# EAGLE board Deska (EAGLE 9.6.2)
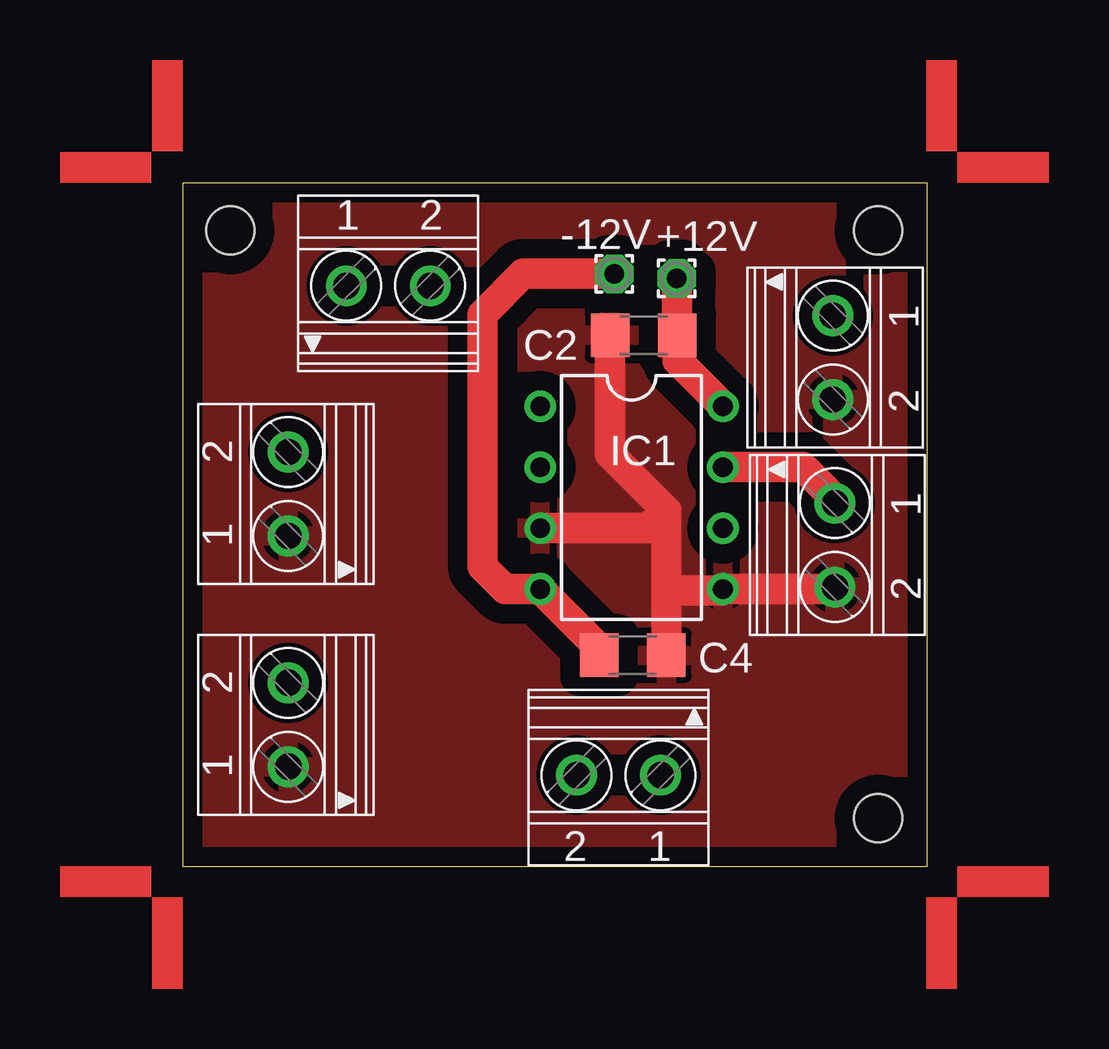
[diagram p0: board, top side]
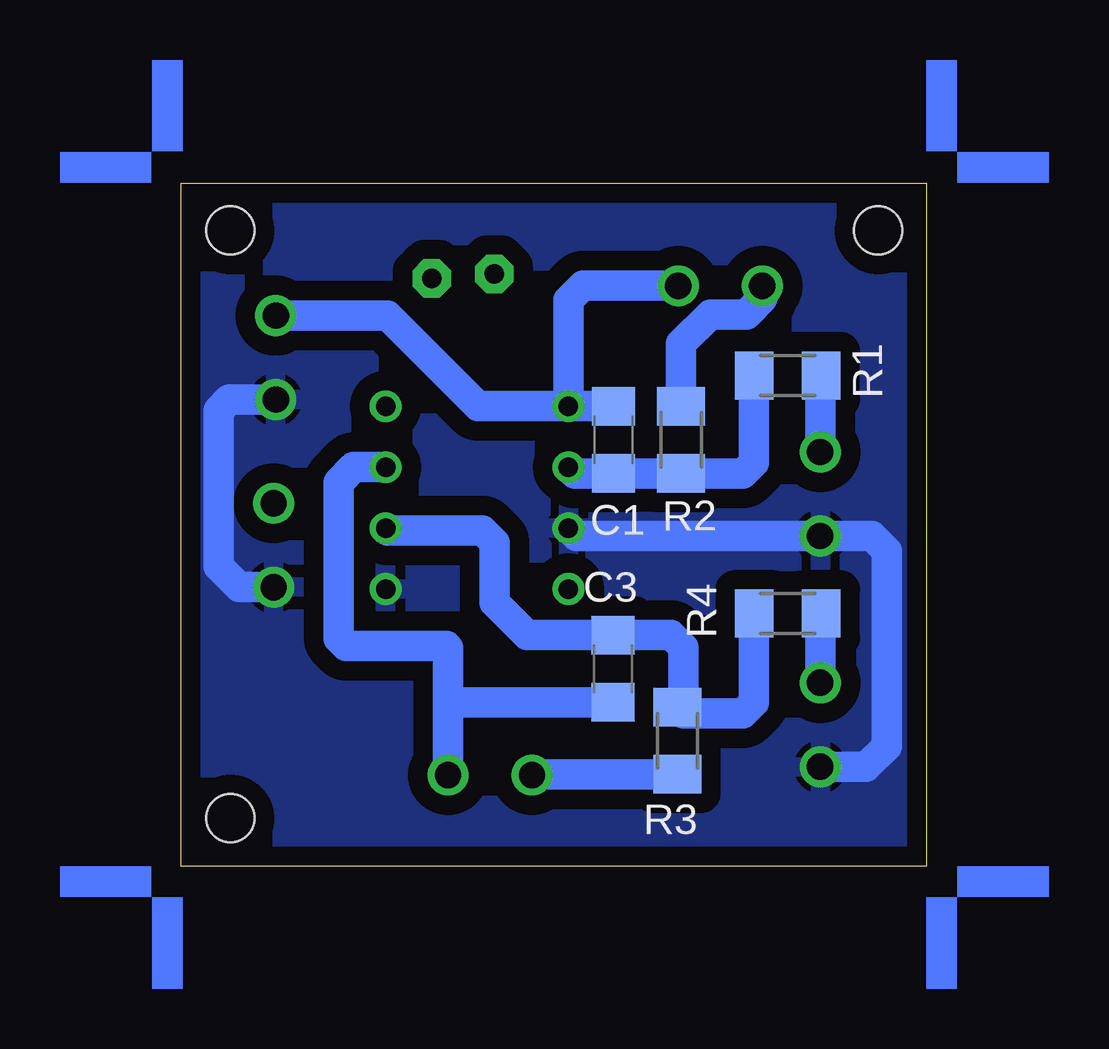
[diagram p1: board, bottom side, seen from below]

Size 31.05 x 28.48 mm. Coordinates in mm from the lower left corner, seen from the top.
Outline: 0,0 31.05,0 31.05,28.48 0,28.48 0,0
Copper layers (1*16): Top 0.035mm / dielectric 1.5mm / Bottom 0.035mm
Design rules "default *": minimum track width 6mil, minimum drill 0.35mm, track to track 6mil, track to pad 6mil, pad to pad 6mil, via to via 6mil, smd to smd 6mil, copper to edge 20mil, drill to drill 6mil, minimum pad ring 10mil, minimum via ring 8mil, stop-mask expansion 4mil, vias tented up to drill 0mil, thermal gap 10mil
Holes 2 mm at 2,26.5 29,2 29,26.5

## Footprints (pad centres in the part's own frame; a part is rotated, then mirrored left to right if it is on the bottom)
1,6/0,8 = drill 0.813 pad 1.6 octagon: 1 0,0
C1206 = smd 1.6 x 1.8: 1 -1.4,0; 2 1.4,0
DIL08 = drill 0.813 pad 1.27: 1 -3.81,-3.81; 2 -1.27,-3.81; 3 1.27,-3.81; 4 3.81,-3.81; 5 3.81,3.81; 6 1.27,3.81; 7 -1.27,3.81; 8 -3.81,3.81
M1206 = smd 1.6 x 2: 1 -1.4,0; 2 1.4,0
1751248 = drill 1.1 pad 1.7: 1 -1.75,-0.1; 2 1.75,-0.1

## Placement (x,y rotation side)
+12V  [1,6/0,8]  20.61,24.5 270 top
-12V  [1,6/0,8]  18,24.69 0 top
C1  [C1206]  13.03,17.77 90 bottom
C2  [C1206]  19.23,22.13 180 top
C3  [C1206]  13.05,8.23 270 bottom
C4  [C1206]  18.77,8.79 0 top
IC1  NE5532  [DIL08]  18.72,15.36 270 top
R1  [M1206]  5.77,20.45 180 bottom
R2  [M1206]  10.21,17.77 90 bottom
R3  [M1206]  10.37,5.23 270 bottom
R4  [M1206]  5.77,10.53 180 bottom
U$1  [ANGLE-SW1-16]  31,28.5 0 top
U$2  [ANGLE-SW1-16]  0,28.5 90 top
U$3  [ANGLE-SW1-16]  0,0 180 top
U$4  [ANGLE-SW1-16]  31,0 270 top
X1  1751248  [1751248]  27.21,21.2 270 top
X2  1751248  [1751248]  27.3,13.38 270 top
X3  1751248  [1751248]  4.31,15.51 90 top
X4  1751248  [1751248]  4.31,5.89 90 top
X5  1751248  [1751248]  8.58,24.29 0 top
X6  1751248  [1751248]  18.18,3.69 180 top

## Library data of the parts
+12V -12V = wirepad
C1-C4 = rcl; SPICEPREFIX: C
IC1 = linear
R1-R4 = rcl; SPICEPREFIX: R
U$1-U$4 = marks
X1-X6 = con-phoenix-350; OC_FARNELL: unknown; OC_NEWARK: unknown

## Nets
+12V: +12V.1 C2.1 IC1.8
-12V: -12V.1 C4.1 IC1.4
GND: C2.2 C4.2 IC1.3 IC1.5 X1.2 X2.2 X3.1 X4.1
N$1: C1.1 IC1.2 R1.2 R2.1
N$2: C3.1 IC1.6 R3.1 R4.2
N$3: R2.2 X5.1
N$4: R3.2 X6.2
N$5: C1.2 IC1.1 X1.1 X5.2
N$6: C3.2 IC1.7 X2.1 X6.1
N$7: R1.1 X3.2
N$8: R4.1 X4.2

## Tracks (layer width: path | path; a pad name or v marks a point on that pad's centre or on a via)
+12V
  Top 1.27: IC1.8 20.63,21.07 C2.1 20.61,22.15 +12V.1
-12V
  Top 1.27: C4.1 17.37,9.09 IC1.4 13.45,11.55 12.5,12.5 12.5,23 14.19,24.69 -12V.1
GND
  Top 1.27: C2.2 17.83,17.17 20.17,14.83 | 20.17,14.83 20.17,11.5 | 20.17,11.5 C4.2 | 20.17,11.5 22.48,11.5 IC1.5 27.12,11.55 X2.2 | IC1.3 19.43,14.09 20.17,14.83
  Bottom 1.27: X4.1 2.5,4.14 1.64,5 1.64,13.14 2.26,13.76 X3.1 14.58,13.76 IC1.3 | X1.2 29.05,19.45 29.5,19 29.5,12.5 28.63,11.63 X2.2
  pour Top (isolate 0.813): 0,0 31,0 31,28.5 0,28.5
  pour Bottom (isolate 0.813): 0,0 31,0 31,28.5 0,28.5
N$1
  Bottom 1.27: R1.2 7.17,16.83 7.63,16.37 R2.1 C1.1 14.65,16.37 IC1.2
N$2
  Bottom 1.27: R4.2 7.17,6.83 7.63,6.37 10.11,6.37 | 10.11,6.37 R3.1 | IC1.6 22.44,14 18.5,14 18,13.5 18,11 16.63,9.63 C3.1 10.63,9.63 10.11,9.11 10.11,6.37
N$3
  Bottom 1.27: R2.2 10.21,21.79 9,23 7.5,23 6.83,23.67 X5.1
N$4
  Bottom 1.27: R3.2 16.39,3.83 X6.2
N$5
  Bottom 1.27: IC1.1 C1.2 | IC1.1 14.91,23.59 14.31,24.19 X5.2 | IC1.1 18.67,19.17 22.45,22.95 X1.1
N$6
  Top 1.27: IC1.7 25.87,16.63 27.2,15.3 X2.1
  Bottom 1.27: IC1.7 23.87,16.63 24.5,16 24.5,9.5 24.17,9.17 20,9.17 19.93,9.1 19.93,7 | X6.1 19.93,7 | C3.2 19.76,6.83 19.93,7
N$7
  Bottom 1.27: X3.2 4.41,20.41 R1.1
N$8
  Bottom 1.27: R4.1 4.41,10.49 X4.2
